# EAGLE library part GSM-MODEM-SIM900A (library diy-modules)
GSM Mini Module based on SIM900A Schematic available here: http://www.electrodragon.com/w/SIM900_(SIM900A)_Mini_DEV_Board
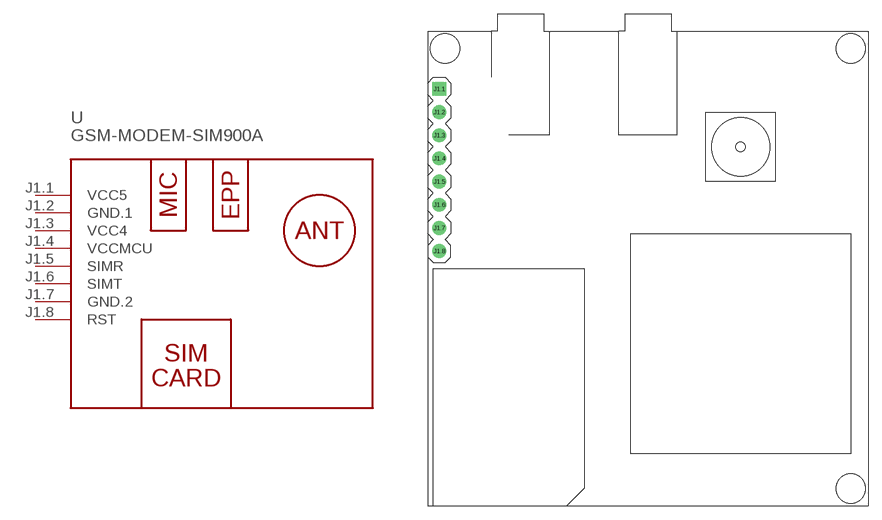
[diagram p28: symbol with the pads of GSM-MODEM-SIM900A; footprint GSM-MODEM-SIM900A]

Designator prefix -

## GSM-MODEM-SIM900A  [GSM-MODEM-SIM900A]
J1.1  VCC5  pwr
J1.2  GND.1  pwr
J1.3  VCC4  pwr
J1.4  VCCMCU  pwr
J1.5  SIMR
J1.6  SIMT
J1.7  GND.2  pwr
J1.8  RST

## Footprint GSM-MODEM-SIM900A (pad centres in mm)
GSM Mini Module based on SIM900A
drill 1 square: J1.1 -22.86,20.32
drill 1: J1.2 -22.86,17.78; J1.3 -22.86,15.24; J1.4 -22.86,12.7; J1.5 -22.86,10.16; J1.6 -22.86,7.62; J1.7 -22.86,5.08; J1.8 -22.86,2.54
hole 3.2 at -22.225,24.765
hole 3.2 at 22.225,24.765
hole 3.2 at 22.225,-23.495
